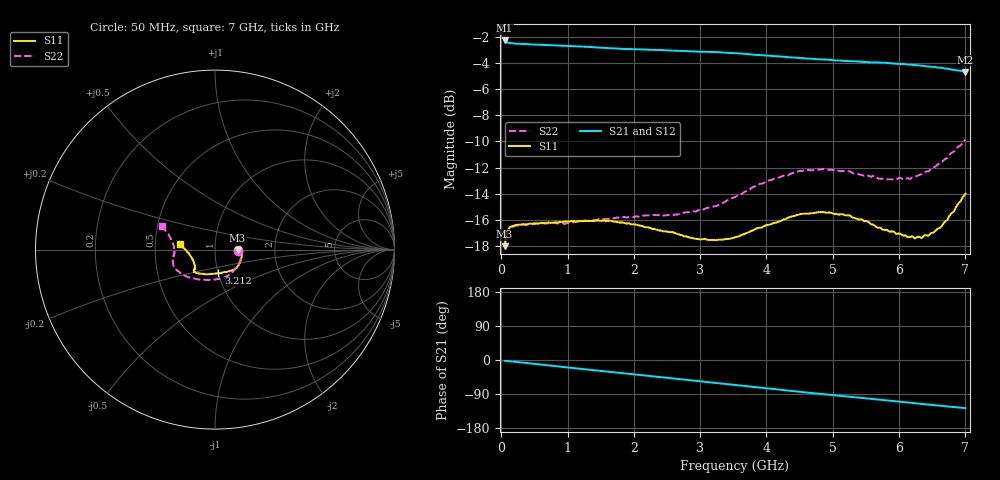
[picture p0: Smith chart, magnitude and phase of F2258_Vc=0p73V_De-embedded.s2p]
! Integrated Device Technology
! Corporate Headquarters
! 6024 Silver Creek Valley Road
! San Jose, CA 95138  USA
! Phone:  1-408-284-8200
! Toll Free:  1-800-223-1366
! Webpage:  http://www.idt.com/
! Timing and RF Division
! 515 Groton Road, Suite 102
! Westford, MA 01886-6024
! Device:  F2258
! Description: Voltage Variable RF Attenuator
! Frequency:  50.0 -  6000.00 MHz
! Package:  3x3 mm Thin QFN Plastic Package: 16 pin
! Ports:  2 RF, 2 DC
!  Pin  1  = NC
!  Pin  2  = NC
!  Pin  3  = RF2  = Port 2
!  Pin  4  = GND
!  Pin  5  = Vdd
!  Pin  6  = NC
!  Pin  7  = VCTRL
!  Pin  8  = NC
!  Pin  9  = GND
!  Pin 10  = RF1  = Port 1
!  Pin 11  = NC
!  Pin 12  = NC
!  Pin 13  = NC
!  Pin 14  = NC
!  Pin 15  = NC
!  Pin 16  = NC
! Vcntrl:  0.730 Volts
! Vdd:  +3.300 Volts
! Current:  1.122 mA
! Data:  The device was measured on a the F2258 evaluation board which has
!  individual transmission lines to the RF pins.  Data was collected
!  using a calibrated network analyzer.  The evaluation board was
!  de-embedded using a TRL calibration technique.
!  The reference plane is the edge of the package pin.
! Misc:  SN 10
!  Action Tracker AT0285
! Date Measured:  2014-12-10
! Date:  2016-01-13  MJV
! Note:
!  Integrated Device Technology supplies this data as a sample of measured
!  data at the package pin for this product.  Your particular data for this
!  product may vary.
!  Data was taken at 25 degrees C.
!  Integrated Device Technology reserves the right to change this data at anytime.
!Freq_(GHz)  S11M_(dB)  S11P_(deg)  S21M_(dB)  S21P_(deg)  S12M_(dB)  S12P_(deg)  S22M_(dB)  S22P_(deg)
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# GHz S dB R 50
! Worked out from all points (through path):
!   201 points, 50 MHz to 7 GHz, reference 50 ohm
!   highest |S21| = -2.28 dB at 50 MHz (marker M1); lowest = -4.7 dB at 7 GHz (marker M2)
!   group delay of S21, straight-line fit = 50.2 ps
!   lowest |S11| = -18.0 dB at 50 MHz (marker M3), VSWR 1.29, Z = 64.4 - j0.562 ohm
!   |S11| at or under -10 dB: start of sweep to end of sweep
!   |S22| runs from -17.9 to -9.9 dB; largest |S21 - S12| = 0.0024
!   S11 on the Smith chart (normalised r, x): 50 MHz: 1.29, -0.01; 3.212 GHz: 1.00, -0.27; 7 GHz: 0.67, +0.05
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0.05  -18.01 -2.0  -2.28 -2.0  -2.29 -2.1  -17.92 -2.4
0.08475  -16.92 -2.9  -2.42 -2.5  -2.43 -2.5  -16.91 -3.7
0.15425  -16.48 -4.6  -2.49 -3.7  -2.51 -3.7  -16.53 -6.6
0.606  -16.22 -17.5  -2.61 -12.2  -2.63 -12.2  -16.26 -23.8
0.9535  -16.13 -28.0  -2.68 -18.8  -2.68 -18.8  -16.32 -38.0
1.2315  -16.10 -34.3  -2.75 -23.9  -2.75 -23.9  -16.08 -47.6
1.6485  -16.06 -42.1  -2.87 -31.5  -2.85 -31.5  -15.88 -60.3
2.37825  -16.80 -55.0  -3.00 -44.7  -3.01 -44.7  -15.62 -80.2
2.58675  -16.93 -59.7  -3.06 -48.5  -3.05 -48.5  -15.66 -86.6
2.93425  -17.45 -70.3  -3.13 -55.0  -3.13 -55.0  -15.35 -99.0
3.21225  -17.55 -81.9  -3.17 -60.2  -3.19 -60.2  -14.97 -109.9
3.525  -17.33 -96.0  -3.25 -66.1  -3.27 -66.1  -14.25 -122.5
4.0115  -16.38 -116.0  -3.43 -75.2  -3.45 -75.2  -13.01 -139.7
4.46325  -15.61 -127.9  -3.61 -83.3  -3.61 -83.3  -12.31 -152.0
4.7065  -15.48 -131.2  -3.68 -87.6  -3.69 -87.5  -12.19 -156.7
5.2625  -15.67 -135.8  -3.87 -97.1  -3.86 -97.1  -12.29 -165.9
5.85325  -16.89 -141.7  -4.02 -107.2  -4.00 -107.2  -12.89 -177.2
6.2355  -17.41 -153.0  -4.15 -113.9  -4.15 -113.9  -12.69 173.9
6.444  -17.20 -162.4  -4.26 -117.6  -4.25 -117.6  -12.29 168.9
6.61775  -16.61 -172.7  -4.36 -120.6  -4.35 -120.6  -11.68 164.2
6.722  -16.03 -177.7  -4.43 -122.5  -4.43 -122.5  -11.29 161.4
7  -14.01 170.6  -4.68 -126.9  -4.67 -126.9  -9.89 156.0
